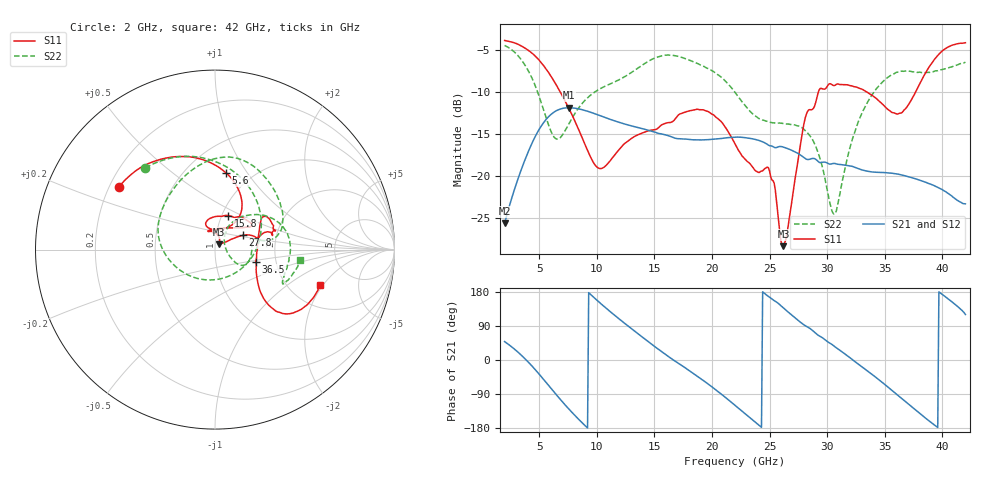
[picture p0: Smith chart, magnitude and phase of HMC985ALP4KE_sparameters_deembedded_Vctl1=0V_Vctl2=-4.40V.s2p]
!s2p File: Measurements: S11, S21, S12, S22
# GHz S dB R 50.0
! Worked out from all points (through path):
!   401 points, 2 GHz to 42 GHz, reference 50 ohm
!   highest |S21| = -11.89 dB at 7.6 GHz (marker M1); lowest = -25.7 dB at 2 GHz (marker M2)
!   lowest |S11| = -28.4 dB at 26.2 GHz (marker M3), VSWR 1.08, Z = 52.3 + j3.17 ohm
!   |S11| at or under -10 dB: 6.821 GHz to 29.25 GHz (22.43 GHz wide, 124 % of centre); 33.42 GHz to 37.69 GHz (4.269 GHz wide, 12 % of centre)
!   |S22| runs from -24.6 to -4.5 dB; largest |S21 - S12| = 0.00024
!   S11 on the Smith chart (normalised r, x): 2 GHz: 0.24, +0.28; 5.6 GHz: 0.76, +0.80; 15.8 GHz: 1.07, +0.42; 27.8 GHz: 1.34, +0.22; 36.5 GHz: 1.57, -0.23; 42 GHz: 2.94, -1.89
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2  -3.88 147.0  -25.66 48.6  -25.67 48.6  -4.47 130.5
3.6  -4.66 120.3  -18.70 8.4  -18.70 8.4  -6.48 84.9
4.7  -5.80 99.5  -15.21 -26.8  -15.21 -26.8  -9.42 43.3
5.6  -7.28 81.9  -13.29 -59.1  -13.30 -59.1  -13.06 -3.8
6.5  -9.22 66.5  -12.25 -92.0  -12.25 -92.0  -15.62 -69.0
7.6  -12.03 54.8  -11.89 -130.1  -11.90 -130.1  -13.76 -135.8
8.7  -15.38 55.0  -12.12 -164.7  -12.12 -164.7  -11.44 -170.3
10.4  -19.13 89.6  -12.90 147.5  -12.90 147.5  -9.56 162.4
15.4  -14.22 75.7  -14.97 27.4  -14.97 27.4  -5.80 87.0
15.8  -13.83 68.7  -15.07 18.5  -15.07 18.5  -5.66 82.0
19.4  -12.23 33.3  -15.71 -57.4  -15.72 -57.4  -7.06 34.9
22  -16.18 51.1  -15.40 -119.6  -15.41 -119.6  -10.07 9.9
24.9  -19.04 104.7  -16.35 167.7  -16.35 167.7  -13.57 13.2
26.2  -28.38 52.7  -16.58 137.3  -16.59 137.3  -13.78 -2.6
27.8  -15.23 27.2  -17.65 96.8  -17.64 96.8  -14.27 -24.6
28.7  -12.11 12.6  -17.94 78.7  -17.95 78.7  -15.62 -31.6
30.6  -9.26 19.5  -18.52 36.8  -18.52 36.8  -24.56 15.5
32.8  -9.59 33.9  -19.19 -13.2  -19.20 -13.2  -13.22 53.2
35.4  -12.21 11.7  -19.66 -74.5  -19.66 -74.5  -8.17 21.3
36.5  -12.47 -16.7  -19.91 -102.3  -19.91 -102.3  -7.54 7.2
39.5  -5.86 -43.7  -21.31 -175.8  -21.31 -175.8  -7.49 -26.3
42  -4.16 -18.6  -23.34 120.1  -23.35 120.0  -6.46 -7.1
